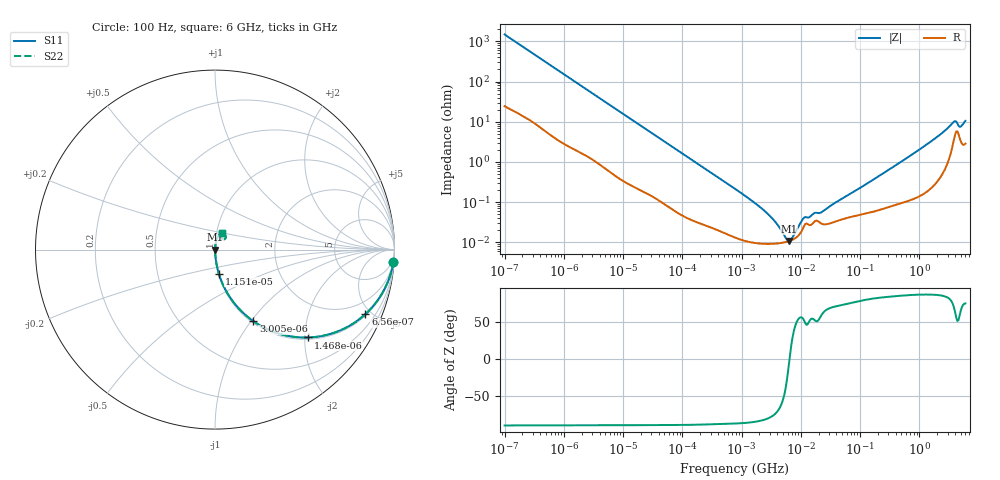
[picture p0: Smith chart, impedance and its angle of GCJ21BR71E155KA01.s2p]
!Murata Part Number: GCJ21BR71E155KA01
!These Parameters are Measured in Series Mode Connection
!Data Generated on Mar 13, 2026
!  o--ll--o
!Port1  Port2
!  o------o
!Operation Temp=25[degC], DC Bias Voltage=0[V]
!Freq. Start=100[Hz] Stop=6[GHz] 401[Steps]
# Hz S RI R 50
!Freq.(Hz) S11(Real) S11(Imag) S21(Real) S21(Imag) S12(Real) S12(Imag) S22(Real) S22(Imag)
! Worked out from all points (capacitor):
!   401 points, 100 Hz to 6 GHz, reference 50 ohm
!   read as one part in series: C = 1.07 uF near 109 Hz
!   lowest |Z| = 10.8 mohm at 6.353 MHz (marker M1)
!   series resonance near 6.458 MHz, so ESL is about 570 pH
!   S11 on the Smith chart (normalised r, x): 100 Hz: 1, -30; 656 Hz: 1.08, -4.62; 1.468 kHz: 1.04, -2.08; 3.005 kHz: 1.02, -1.03; 11.51 kHz: 1.01, -0.27; 6 GHz: 1.06, +0.20
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100  0.9944 -0.0671  0.00564 0.0671  0.00564 0.0671  0.9944 -0.0671
320  0.9529 -0.2024  0.0471 0.2024  0.0471 0.2024  0.9529 -0.2024
656  0.8377 -0.3597  0.1623 0.3597  0.1623 0.3597  0.8377 -0.3597
1468  0.5193 -0.4897  0.4807 0.4897  0.4807 0.4897  0.5193 -0.4897
2008  0.371 -0.4725  0.629 0.4725  0.629 0.4725  0.371 -0.4725
3005  0.214 -0.3991  0.786 0.3991  0.786 0.3991  0.214 -0.3991
5378  0.0823 -0.2641  0.9177 0.2641  0.9177 0.2641  0.0823 -0.2641
11514  0.0211 -0.1332  0.9789 0.1332  0.9789 0.1332  0.0211 -0.1332
40335  0.00267 -0.0396  0.9973 0.0396  0.9973 0.0396  0.00267 -0.0396
774597  0.000136 -0.00215  0.9999 0.00215  0.9999 0.00215  0.000136 -0.00215
2713602  9.2e-05 -0.00052  0.9999 0.00052  0.9999 0.00052  9.2e-05 -0.00052
5809218  0.000104 -5.73e-05  0.9999 5.73e-05  0.9999 5.73e-05  0.000104 -5.73e-05
6353432  0.000108 -8.8e-06  0.9999 8.8e-06  0.9999 8.8e-06  0.000108 -8.8e-06
7266822  0.000117 6.53e-05  0.9999 -6.53e-05  0.9999 -6.53e-05  0.000117 6.53e-05
1.087309e7  0.000224 0.000309  0.9998 -0.000309  0.9998 -0.000309  0.000224 0.000309
1.555665e7  0.000287 0.000395  0.9997 -0.000395  0.9997 -0.000395  0.000287 0.000395
2.327686e7  0.000286 0.00051  0.9997 -0.00051  0.9997 -0.00051  0.000286 0.00051
3.124326e8  0.000806 0.00649  0.9992 -0.00649  0.9992 -0.00649  0.000806 0.00649
1.637704e9  0.00345 0.0335  0.9965 -0.0335  0.9965 -0.0335  0.00345 0.0335
3.666503e9  0.0328 0.0849  0.9672 -0.0849  0.9672 -0.0849  0.0328 0.0849
5.016141e9  0.0358 0.064  0.9642 -0.064  0.9642 -0.064  0.0358 0.064
6e9  0.037 0.0948  0.963 -0.0948  0.963 -0.0948  0.037 0.0948
